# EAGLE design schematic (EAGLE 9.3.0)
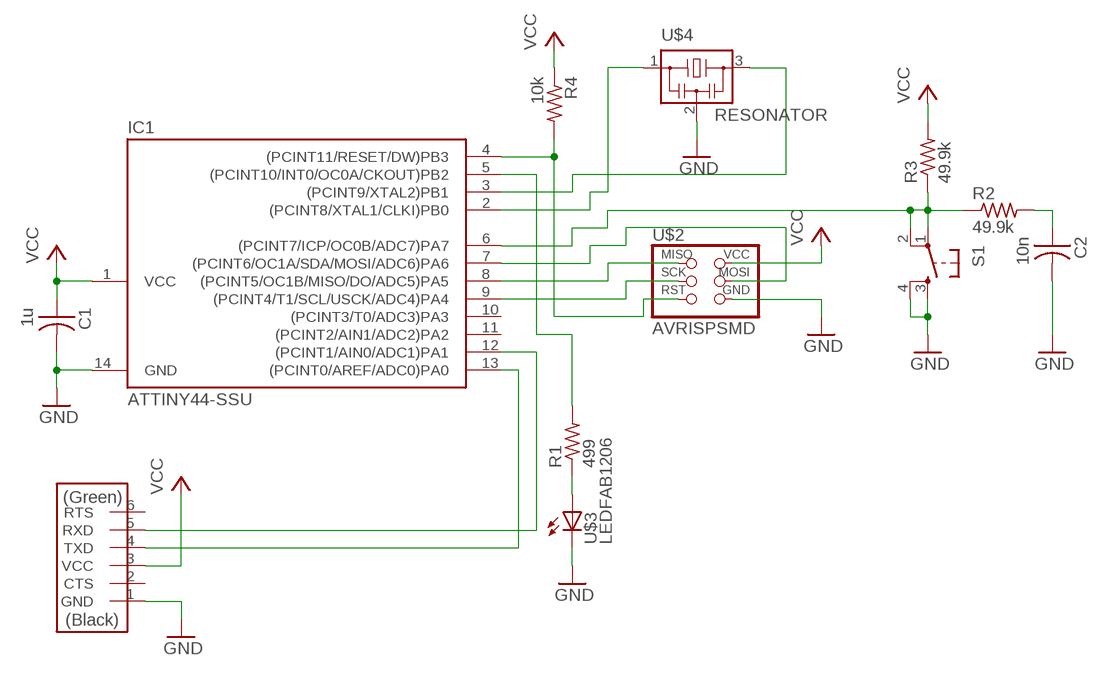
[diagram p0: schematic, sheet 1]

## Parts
C1  1u  CAP-US1206FAB  [C1206FAB]
C2  10n  CAP-US1206FAB  [C1206FAB]
IC1  ATTINY44-SSU  [SOIC14]
R1  499  RES-US1206FAB  [R1206FAB]
R2  49.9k  RES-US1206FAB  [R1206FAB]
R3  49.9k  RES-US1206FAB  [R1206FAB]
R4  10k  RES-US1206FAB  [R1206FAB]
S1  6MM_SWITCH6MM_SWITCH  [6MM_SWITCH]
U$1  FTDI-SMD-HEADER  [1X06SMD]
U$2  AVRISPSMD  [2X03SMD]
U$3  LEDFAB1206  [LED1206FAB]
U$4  RESONATOR  [EFOBM]

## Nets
GND: C1.2 C2.2 IC1.14(GND) S1.3(S) S1.4(S1) U$1.1(GND) U$2.6(GND) U$3.2(C) U$4.2
N$1: IC1.4((PCINT11/RESET/DW)PB3) R4.2 U$2.5(RST)
N$2: IC1.2((PCINT8/XTAL1/CLKI)PB0) U$4.1
N$3: IC1.3((PCINT9/XTAL2)PB1) U$4.3
N$4: IC1.6((PCINT7/ICP/OC0B/ADC7)PA7) R2.1 R3.1 S1.1(P) S1.2(P1)
N$5: C2.1 R2.2
N$6: IC1.8((PCINT5/OC1B/MISO/DO/ADC5)PA5) U$2.1(MISO)
N$7: IC1.9((PCINT4/T1/SCL/USCK/ADC4)PA4) U$2.3(SCK)
N$8: R1.1 U$3.1(A)
N$9: IC1.7((PCINT6/OC1A/SDA/MOSI/ADC6)PA6) U$2.4(MOSI)
N$10: IC1.5((PCINT10/INT0/OC0A/CKOUT)PB2) R1.2
N$11: IC1.12((PCINT1/AIN0/ADC1)PA1) U$1.5(RXD)
N$13: IC1.13((PCINT0/AREF/ADC0)PA0) U$1.4(TXD)
VCC: C1.1 IC1.1(VCC) R3.2 R4.1 U$1.3(VCC) U$2.2(VCC)
Unconnected: IC1.10((PCINT3/T0/ADC3)PA3) IC1.11((PCINT2/AIN1/ADC2)PA2) U$1.2(CTS) U$1.6(RTS)

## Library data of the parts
C1 C2 = eagle_fab:CAP-US
IC1 = eagle_fab:ATTINY44
R1-R4 = eagle_fab:RES-US: Resistor (US Symbol)
S1 = eagle_fab:6MM_SWITCH: OMRON SWITCH
U$1 = eagle_fab:FTDI-SMD-HEADER
U$2 = eagle_fab:AVRISP
U$3 = eagle_fab:LED: LED
U$4 = eagle_fab:RESONATOR

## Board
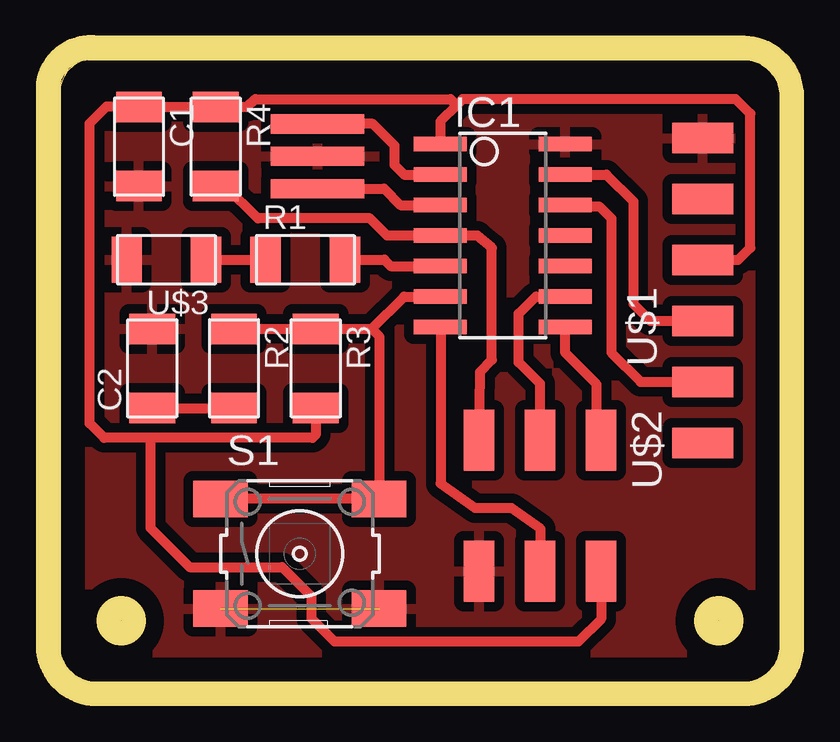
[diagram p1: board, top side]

Size 29.98 x 25.91 mm. Coordinates in mm from the lower left corner, seen from the top.
Outline: 1.16,0 28.84,0 arc90 29.98,1.14 29.98,24.77 arc90 28.84,25.91 1.16,25.91 arc90 0.01,24.38 0.01,1.14 arc90 1.16,0
Copper layers (1*16): Top 0.035mm / dielectric 1.5mm / Bottom 0.035mm
Design rules "default *": minimum track width 16mil, minimum drill 0.35mm, track to track 16mil, track to pad 16mil, pad to pad 16mil, via to via 16mil, smd to smd 16mil, copper to edge 40mil, drill to drill 6mil, minimum pad ring 10mil, minimum via ring 8mil, stop-mask expansion 4mil, vias tented up to drill 0mil, thermal gap 16mil
Holes 1.52 mm at 27.44,2.54 2.55,2.54
Milling: area 2,2 to 3.1,3; area 26.9,2 to 28,3; 8 lines

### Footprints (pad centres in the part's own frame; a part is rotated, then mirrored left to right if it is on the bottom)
C1206FAB = smd 1.27 x 1.905: 1 -1.651,0; 2 1.651,0
SOIC14 = smd 0.61 x 2.21: 1 -3.81,-2.603; 2 -2.54,-2.603; 3 -1.27,-2.603; 4 0,-2.603; 5 1.27,-2.603; 6 2.54,-2.603; 7 3.81,-2.603; 8 3.81,2.603; 9 2.54,2.603; 10 1.27,2.603; 11 0,2.603; 12 -1.27,2.603; 13 -2.54,2.603; 14 -3.81,2.603
R1206FAB = smd 1.27 x 1.905: 1 -1.651,0; 2 1.651,0
6MM_SWITCH = smd 2.286 x 1.524: 1 -3.302,2.286; 2 3.302,2.286; 3 -3.302,-2.286; 4 3.302,-2.286
1X06SMD = smd 2.54 x 1.27: 1 0,6.35; 2 0,3.81; 3 0,1.27; 4 0,-1.27; 5 0,-3.81; 6 0,-6.35
2X03SMD = smd 2.54 x 1.27: 1 -2.54,2.54; 2 2.92,2.54; 3 -2.54,0; 4 2.92,0; 5 -2.54,-2.54; 6 2.92,-2.54
LED1206FAB = smd 1.27 x 1.905: 1 -1.651,0; 2 1.651,0
EFOBM = smd 0.8 x 3.9: 1 -1.35,0; 2 0,0; 3 1.35,0

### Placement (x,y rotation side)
C1  3.29,22.3 270 top
C2  3.84,13.06 90 top
IC1  18.45,18.59 270 top
R1  10.22,17.59 0 top
R2  7.25,13.06 270 top
R3  10.65,13.06 270 top
R4  6.49,22.3 270 top
S1  9.99,5.33 0 top
U$1  26.78,16.31 0 top
U$2  20,7.52 270 top
U$3  4.43,17.59 180 top
U$4  10.73,21.89 270 top

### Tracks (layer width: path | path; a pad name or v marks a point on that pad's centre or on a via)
GND  (1 unrouted)
  pour Top (isolate 0.406): 0.01,0 30.39,0 30.39,26.75 0.01,26.75
N$1
  Top 0.406: R4.2 6.9,20.65 8.24,19.3 12.92,19.3 13.63,18.59 IC1.4 17.39,18.59 18,18.09 18,13.41 17.5,12.92 U$2.5
N$2
  Top 0.406: IC1.2 14.34,21.13 13.93,21.54 13.93,22.35 13.04,23.25 U$4.1
N$3
  Top 0.406: U$4.3 13.5,20.55 14.19,19.86 IC1.3
N$4
  Top 0.406: S1.1 S1.2 13.32,7.65 13.32,14.38 12.99,14.71 | IC1.6 14.34,16.05 12.99,14.71 | R2.1 R3.1 12.99,14.71
N$5
  Top 0.406: C2.1 R2.2
N$6
  Top 0.406: U$2.1 22.36,10.24 22.36,12.39 21.06,13.7 IC1.8
N$7
  Top 0.406: IC1.9 19.82,16.05 19.11,15.34 19.11,13.31 20,12.42 U$2.3
N$8
  Top 0.406: U$3.1 R1.1
N$9
  Top 0.406: U$2.4 20.02,6.37 18.82,7.23 17.3,7.23 15.86,8.26 IC1.7
N$10
  Top 0.406: R1.2 13.52,17.59 13.78,17.32 IC1.5
N$11
  Top 0.406: IC1.12 21.11,19.81 22.47,19.81 22.97,19.3 22.97,13.72 24.19,12.5 U$1.5
N$13
  Top 0.406: IC1.13 22.77,21.13 23.89,20.02 23.89,15.75 24.6,15.04 U$1.4
VCC
  Top 0.406: IC1.1 15.85,23.36 16.52,24.03 | 16.52,24.03 16.78,24.28 28.16,24.28 28.77,23.67 28.77,18.09 28.26,17.58 U$1.3 | 16.52,24.03 16.27,24.28 8.14,24.28 7.81,23.95 R4.1 3.57,23.95 | C1.1 3.57,23.95 | R3.2 10.66,10.29 10.53,10.16 3.77,10.16 | 3.57,23.95 3.54,23.98 1.94,23.98 1.23,23.27 1.23,10.77 1.84,10.16 3.77,10.16 | U$2.2 22.54,2.62 21.6,1.68 11.44,1.68 10.48,2.64 10.48,3.56 9.26,4.78 5.4,4.78 3.77,6.4 3.77,10.16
